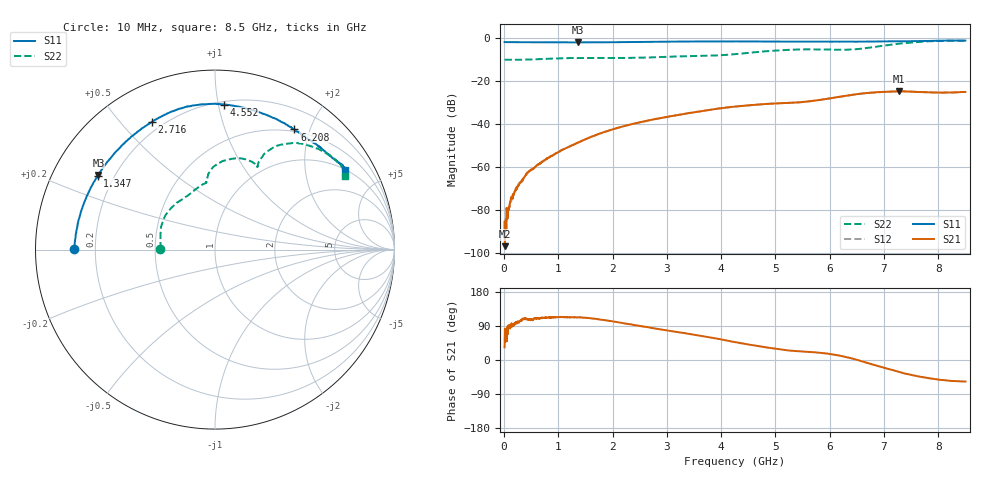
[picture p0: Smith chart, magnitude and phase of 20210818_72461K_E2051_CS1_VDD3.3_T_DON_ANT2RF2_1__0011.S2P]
!Agilent Technologies,E5071C,MY46417908,A.11.23
!Date: Wed Aug 18 14:27:43 2021
!Data & Calibration Information:
!Freq	S11:SOLT2(ON)	S21:SOLT2(ON)	S12:SOLT2(ON)	S22:SOLT2(ON)
!PortZ  Port1:50+j0  Port2:50+j0
!Above PortZ is port z conversion or system Z0 setting when saving the data.
!When reading, reference impedance value at option line is always used.
# Hz S dB R 50
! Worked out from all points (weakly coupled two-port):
!   1601 points, 10 MHz to 8.5 GHz, reference 50 ohm
!   highest |S21| = -24.95 dB at 7.269 GHz (marker M1); lowest = -96.8 dB at 15.31 MHz (marker M2)
!   lowest |S11| = -2.3 dB at 1.368 GHz (marker M3), VSWR 7.75, Z = 7 + j14.4 ohm
!   |S11| at or under -10 dB: nowhere
!   |S22| runs from -10.3 to -1.5 dB; largest |S21 - S12| = 0.00027
!   S11 on the Smith chart (normalised r, x): 10 MHz: 0.12, +0.00; 1.347 GHz: 0.14, +0.28; 2.716 GHz: 0.16, +0.61; 4.552 GHz: 0.22, +1.04; 6.208 GHz: 0.47, +1.76; 8.5 GHz: 1.00, +3.24
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1e7  -2.09 179.7  -85.53 33.5  -88.79 21.1  -10.29 179.6
1.530625e7  -2.11 179.6  -96.85 82.4  -84.42 54.2  -10.30 179.5
6.30625e7  -2.13 178.5  -84.08 67.2  -82.82 82.7  -10.32 178.5
1.798e8  -2.15 175.9  -73.06 94.3  -72.19 97.4  -10.34 175.6
2.275562e8  -2.16 174.7  -70.61 97.8  -70.40 96.7  -10.33 174.6
4.451125e8  -2.18 169.7  -62.40 106.4  -62.37 105.0  -10.22 170.1
8.1655e8  -2.22 160.9  -55.87 111.8  -55.86 111.8  -9.86 160.4
1.347175e9  -2.24 147.9  -48.97 112.3  -48.99 112.5  -9.47 144.2
1.3684e9  -2.26 147.4  -48.73 112.5  -48.65 112.8  -9.48 143.6
1.426769e9  -2.24 145.9  -48.02 112.2  -48.05 112.0  -9.46 141.8
1.994538e9  -2.18 131.8  -42.67 102.1  -42.69 102.0  -9.51 125.8
2.716188e9  -2.01 116.3  -38.18 84.7  -38.20 84.6  -9.23 110.6
2.843538e9  -1.97 114.2  -37.58 81.7  -37.58 81.7  -9.09 108.7
4.255e9  -1.81 91.8  -32.08 47.3  -32.07 47.4  -7.72 95.6
4.55215e9  -1.84 86.6  -31.39 39.8  -31.42 39.9  -7.02 92.7
5.671769e9  -1.90 65.0  -29.47 20.9  -29.49 21.0  -5.50 68.9
6.2077e9  -1.91 56.6  -27.37 10.8  -27.39 10.7  -5.68 63.1
6.679956e9  -1.89 50.1  -25.78 -7.1  -25.81 -7.2  -4.90 63.2
7.088538e9  -1.78 45.5  -25.10 -24.0  -25.12 -24.1  -3.43 59.2
7.26895e9  -1.74 43.6  -24.95 -31.1  -24.97 -31.2  -2.87 55.4
7.937538e9  -1.52 36.1  -25.51 -50.4  -25.50 -50.4  -1.62 39.0
8.5e9  -1.40 31.6  -25.26 -56.8  -25.27 -57.0  -1.58 29.6
